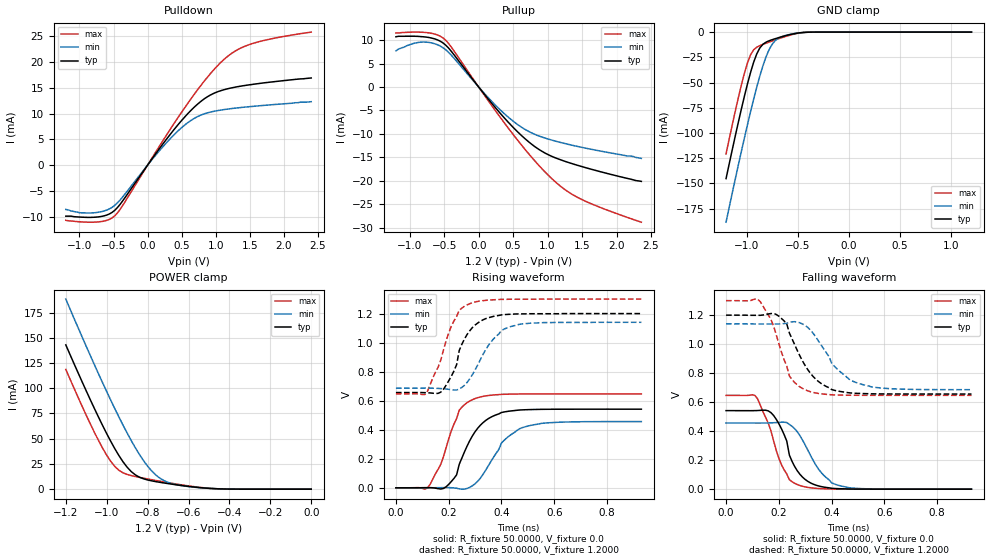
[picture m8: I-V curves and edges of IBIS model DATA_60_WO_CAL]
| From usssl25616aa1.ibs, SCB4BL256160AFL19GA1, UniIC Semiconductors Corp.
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|   Model DATA_60_WO_CAL
[Model]  DATA_60_WO_CAL
Model_type I/O
Polarity   Non-Inverting
Enable   Active-High
Vinl =   0.3800V
Vinh =   0.8200V
Vmeas =  0.6000V
Cref =   5.0000pF
Rref =   50.0000
Vref =   0.6000V
C_comp   1.7430pF   1.7110pF   1.7640pF
[Temperature Range]   25.0000   0.1250k   -40.0000
[Voltage Range]   1.2000V   1.1400V   1.3000V
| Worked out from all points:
|   slope of the pulldown table from 0 to 0.18 V, typ, clamps not added: 54.2 ohm
|   slope of the pullup table from 0 to 0.18 V, typ, clamps not added: 54.6 ohm
|   GND clamp passes 1 mA (typ) near -0.50 V on its own axis
|   POWER clamp passes 1 mA (typ) near -0.51 V on its own axis
|   rising waveform, R_fixture 50.0000, V_fixture 0.0: 20-80 % time 88.7ps typ, 106ps min, 76.6ps max; typ from 0 V to 0.542 V
|   rising waveform, R_fixture 50.0000, V_fixture 1.2000: 20-80 % time 75.5ps typ, 94.4ps min, 81.4ps max; typ from 0.656 V to 1.2 V
|   falling waveform, R_fixture 50.0000, V_fixture 0.0: 20-80 % time 72.3ps typ, 91.5ps min, 77.3ps max; typ from 0.542 V to 0 V
|   falling waveform, R_fixture 50.0000, V_fixture 1.2000: 20-80 % time 98.8ps typ, 115ps min, 71ps max; typ from 1.2 V to 0.656 V
[Pulldown]
|Voltage   I(typ)   I(min)   I(max)
-1.2V     -9.9mA     -8.6mA     -10.7mA
-800mV    -10.12mA   -9.26mA    -11.07mA
-600mV    -9.689mA   -8.724mA   -10.72mA
-480mV    -8.742mA   -7.783mA   -9.813mA
-360mV    -6.833mA   -6.077mA   -7.71mA
200mV     3.678mA    3.203mA    4.233mA
520mV     8.97mA     7.504mA    10.66mA
840mV     12.94mA    9.985mA    16.44mA
1.2V      14.89mA    10.91mA    21.36mA
1.36V     15.3mA     11.16mA    22.66mA
1.6V      15.77mA    11.46mA    23.82mA
2.4V      16.9mA     12.3mA     25.8mA
[Pullup]
|Voltage   I(typ)   I(min)   I(max)
-1.2V     10.7mA     7.7mA      11.5mA
-840mV    10.73mA    9.55mA     11.67mA
-680mV    10.41mA    9.372mA    11.42mA
-520mV    9.417mA    8.392mA    10.48mA
-400mV    7.656mA    6.82mA     8.572mA
80mV      -1.49mA    -1.327mA   -1.686mA
360mV     -6.382mA   -5.519mA   -7.39mA
600mV     -10.04mA   -8.356mA   -11.97mA
840mV     -12.96mA   -10.24mA   -16.16mA
1.12V     -15.13mA   -11.55mA   -20.3mA
1.4V      -16.53mA   -12.55mA   -23.23mA
2.36V     -20.1mA    -15.2mA    -28.79mA
[GND_clamp]
|Voltage   I(typ)   I(min)   I(max)
-1.2V     -145.3mA   -188.5mA   -120.8mA
-1.05V    -76.2mA    -118.2mA   -52.43mA
-990mV    -51.2mA    -91.62mA   -30.39mA
-960mV    -39.9mA    -78.82mA   -22.48mA
-900mV    -21.67mA   -54.7mA    -15mA
-870mV    -15.78mA   -43.66mA   -13.45mA
-810mV    -10.04mA   -24.79mA   -11.07mA
-780mV    -8.658mA   -17.59mA   -9.958mA
-720mV    -6.57mA    -8.545mA   -7.793mA
-630mV    -3.906mA   -3.64mA    -4.741mA
-420mV    -215.4uA   -240.5uA   -235uA
1.2V      1.597nA    22.84nA    1.463nA
[POWER_clamp]
|Voltage   I(typ)   I(min)   I(max)
-1.2V     143mA      188.4mA    118.7mA
-1.1V     97.38mA    141.5mA    73.24mA
-1.04V    71.38mA    114.3mA    48.22mA
-1V       55.04mA    96.69mA    33.64mA
-960mV    40mA       79.65mA    22.42mA
-900mV    21.75mA    55.6mA     14.58mA
-860mV    14.17mA    41.05mA    12.52mA
-800mV    9.133mA    22.79mA    10.12mA
-740mV    6.786mA    10.88mA    7.886mA
-660mV    4.332mA    4.436mA    5.101mA
-520mV    1.103mA    1.063mA    1.274mA
0V        1.597nA    6.003nA    2.16nA
[Ramp]
| variable   typ   min   max
dV/dt_r  0.3250/88.8406p   0.2738/0.1075n   0.3881/77.1250p
dV/dt_f  0.3264/93.6061p   0.2723/0.1179n   0.3917/75.3477p
R_load = 50.0000
[Rising Waveform]
R_fixture= 50.0000
V_fixture= 0.0
V_fixture_min= 0.0
V_fixture_max= 0.0
|time   V(typ)   V(min)   V(max)
0s        0V         0V         0V
120ps     1.169mV    174.2uV    -632.8uV
170ps     -8.318mV   1.001mV    162.2mV
220ps     64.7mV     -906.8uV   439.1mV
240ps     162.2mV    -7.625mV   534.8mV
300ps     386.3mV    27.88mV    614.6mV
400ps     518.7mV    308.3mV    643.6mV
470ps     536mV      408.3mV    646.2mV
590ps     541mV      449.1mV    646.8mV
930ps     541.6mV    456.3mV    646.8mV
[Rising Waveform]
R_fixture= 50.0000
V_fixture= 1.2000
V_fixture_min= 1.1400
V_fixture_max= 1.3000
|time   V(typ)   V(min)   V(max)
0s        656mV      686mV      647.1mV
110ps     655.3mV    686.5mV    642.9mV
170ps     658.9mV    683.4mV    879.8mV
220ps     805mV      673.7mV    1.15V
230ps     848.4mV    673.1mV    1.18V
240ps     946.5mV    681.2mV    1.223V
280ps     1.082V     751.1mV    1.268V
360ps     1.176V     1.004V     1.294V
430ps     1.195V     1.108V     1.299V
930ps     1.2V       1.14V      1.3V
[Falling Waveform]
R_fixture= 50.0000
V_fixture= 0.0
V_fixture_min= 0.0
V_fixture_max= 0.0
|time   V(typ)   V(min)   V(max)
0s        541.6mV    456.3mV    646.8mV
110ps     541.7mV    455.9mV    645.6mV
160ps     539.8mV    456.8mV    454.9mV
180ps     508.7mV    458.1mV    334.5mV
230ps     331.8mV    459.6mV    105.2mV
240ps     234.8mV    446mV      65.31mV
270ps     126.6mV    395.6mV    31.85mV
350ps     22.47mV    139.4mV    4.671mV
420ps     3.913mV    29.76mV    683.3uV
930ps     0V         0V         0V
[Falling Waveform]
R_fixture= 50.0000
V_fixture= 1.2000
V_fixture_min= 1.1400
V_fixture_max= 1.3000
|time   V(typ)   V(min)   V(max)
0s        1.2V       1.14V      1.3V
130ps     1.199V     1.139V     1.292V
170ps     1.211V     1.139V     1.171V
230ps     1.14V      1.144V     848.6mV
250ps     1.037V     1.154V     756mV
310ps     823.2mV    1.115V     677.8mV
400ps     687mV      869.4mV    650.7mV
490ps     661.4mV    737.3mV    647.5mV
610ps     656.6mV    694.5mV    647.1mV
930ps     656mV      686.1mV    647.1mV
